FUNCTION_BLOCK "IMAC_VALVE"
TITLE = VALVE
//--------------------------------------------------------------------------------
//SIEMENS AG     I&S IP PEP SN                       PSP-Element: D-09300081-E-E5
//--------------------------------------------------------------------------------
//History
//=======
//Date       Version Description                     Author
//1997/06/09   0.6   Basic EditionHeino              Salge
//2004/11/05   1.0   Basic Edition converted to S7   Edelmann
//2004/12/07   1.1   Interface adapted               Edelmann
//2004/12/16   1.2   ACOM converted to WORD          Edelmann
//
//--------------------------------------------------------------------------------
//PLC:   >= S7-300
//--------------------------------------------------------------------------------
//Specification:   Refer "TECHFUNK.DOC"
//--------------------------------------------------------------------------------
//Called FC: FC90 "DELAYTIMER"
//           SFC20 "BLKMOV"
//--------------------------------------------------------------------------------
//at run time:
//--------------------------------------------------------------------------------
//
//--------------------------------------------------------------------------------
//Note:
//--------------------------------------------------------------------------------
// KNOW_HOW_PROTECT
AUTHOR : Sa_Edm
FAMILY : IMAC
NAME : VALVE
VERSION : 1.2


VAR_INPUT
  OBJ : INT ;
  RMOT : BOOL ;	//Local / Remote
  OPEN : BOOL ;
  CLSD : BOOL ;
  ACOM : WORD ;
  FAUL : BOOL ;
  PCONF : STRUCT
   LastRecord : INT  := 100;
   Pointer1stRecord : STRUCT
    S7ID : BYTE  := B#16#10;	//ANY pointer: ID S7
    Typ : BYTE  := B#16#2;	//ANY pointer: data typ =02 BYTE =04 WORD =05 INT =06 DWORD =07 DINT =08 REAL
    RepeatFactor : INT  := 104;	//ANY pointer: repeat factor
    DBNo : INT  := 83;	//ANY pointer: DB number, zero if no DB
    MemoryArea : BYTE  := B#16#84;	//ANY pointer: Memory area =81 IN =82 OUT =83 M =84 DB =85 DI =86 L
    DWHigh : BYTE ;	//ANY pointer: DW highest byte
    DWX : INT ;	//ANY pointer: DW low / bit (address = byte *8 + bit)
   END_STRUCT ;
  END_STRUCT ;
END_VAR
VAR_OUTPUT
  VOPN : BOOL ;
  VCLS : BOOL ;
  STAT : WORD ;
  OSSTAT : WORD ;	//Status for OS
  OSALARM : WORD ;	//Alarms for OS
END_VAR
VAR_IN_OUT
  OSCOM : WORD ;
END_VAR
VAR
  VALVE : STRUCT
   System : WORD ;
   CmdOS : WORD ;
   MirrorCmdOS : WORD ;
   Test : WORD ;
   AlarmOS : WORD ;
   StatusOS : WORD ;
   SysStatusOS : WORD ;
   Status1 : WORD ;
   Status2 : WORD ;
   Status3 : BYTE ;
   InputEdges : BYTE ;
   AutoEdges : WORD ;
   DataTimeActFault : STRUCT
    StartTime : DINT ;
    StartEdge : BOOL ;
   END_STRUCT ;
   DataTimeOpening : STRUCT
    StartTime : DINT ;
    StartEdge : BOOL ;
   END_STRUCT ;
   DataTimeClosing : STRUCT
    StartTime : DINT ;
    StartEdge : BOOL ;
   END_STRUCT ;
   DataTimeFeedback : STRUCT
    StartTime : DINT ;
    StartEdge : BOOL ;
   END_STRUCT ;
   DataTimeReverse : STRUCT
    StartTime : DINT ;
    StartEdge : BOOL ;
   END_STRUCT ;
   DataTimeOvertravel : STRUCT
    StartTime : DINT ;
    StartEdge : BOOL ;
   END_STRUCT ;
   DataTimeExtFault : STRUCT
    StartTime : DINT ;
    StartEdge : BOOL ;
   END_STRUCT ;
   DataTimeRestart : STRUCT
    StartTime : DINT ;
    StartEdge : BOOL ;
   END_STRUCT ;
   PCONF : STRUCT
    Modeswitches : STRUCT
     M0_SingleActingValve : BOOL ;	// Single acting valve (1); Double acting valve (0)
     M1_ResetMode : BOOL ;	// Open/Close and RESET (1); only RESET (0)
     M2_OperationMode : BOOL ;	// AUTO/MANUAL/LOCAL(1); Only MANUAL/LOCAL
     M3_Status : BOOL ;	// Change status OPENED/CLOSED by switching from REMOTE to LOCAL (1)
     M4_LockInput : BOOL ;	// Commands and failure (1); only failure
     M5_ESO : BOOL ;	// Open valve if ESO=1 (1); Close valve if ESO=1 (0)
     M6_ReverseTime : BOOL ;	// Double acting valves: Reverse Time ON
     M7_OvertravelTime : BOOL ;	// Double acting valves: Overtravel Time ON
     M8_Spare : BOOL ;	// Spare
     M9_OpenAfterBlackout : BOOL ;	// Open after blackout (1)
     M10_ExtFaultNC : BOOL ;	// External Fault is NC (1); NO (0)
     M11_Spare : BOOL ;	// Spare
     M12_Spare : BOOL ;	// Spare
     M13_LocalAutoMode : BOOL ;	// Set automatic status if RMOT-input is in local
     M14_Spare : BOOL ;	// Spare
     M15_Test : BOOL ;	// Testbit (1)
    END_STRUCT ;
    DlyTActFault : TIME ;	// Setpoint Action Fault delay
    DlyTOpening : TIME ;	// Setpoint Waiting Delay Slow->Fast
    DlyTClosing : TIME ;	// Setpoint Waiting Delay Fast->Slow
    DlyTFeedback : TIME ;	// Setpoint feedback fault delay
    DlyTReverse : TIME ;	// Setpoint change direction
    DlyTOvertravel : TIME ;	// Setpoint auto alarm delay
    DlyTExtFault : TIME ;	// Setpoint external fault delay
    DlyTRestart : TIME ;	// Setpoint restart after blackout delay
   END_STRUCT ;
  END_STRUCT ;
  siFailRR : INT ;	//Falure blockmove readrecord
  siFailWR : INT ;	//Failure blokmove write record
END_VAR
VAR_TEMP
  M200_0 : BOOL ;
  tbCmdManual : BOOL ;
  tbCmdAuto : BOOL ;
  M200_3 : BOOL ;
  M200_4 : BOOL ;
  M200_5 : BOOL ;
  M200_6 : BOOL ;
  M200_7 : BOOL ;
  tbOSCmdOpen : BOOL ;
  tbOSCmdClose : BOOL ;
  tbOSCmdTgOpCl : BOOL ;
  M201_3 : BOOL ;
  M201_4 : BOOL ;
  M201_5 : BOOL ;
  M201_6 : BOOL ;
  tbCmdReset : BOOL ;
  M202_0 : BOOL ;
  M202_1 : BOOL ;
  M202_2 : BOOL ;
  M202_3 : BOOL ;
  M202_4 : BOOL ;
  M202_5 : BOOL ;
  M202_6 : BOOL ;
  M202_7 : BOOL ;
  M203_0 : BOOL ;
  M203_1 : BOOL ;
  M203_2 : BOOL ;
  tbLock : BOOL ;
  tbAmergency : BOOL ;
  tbBlackout : BOOL ;
  tb24VPleiger : BOOL ;
  M203_7 : BOOL ;
  M204_0 : BOOL ;
  M204_1 : BOOL ;
  M204_2 : BOOL ;
  M204_3 : BOOL ;
  M204_4 : BOOL ;
  M204_5 : BOOL ;
  M204_6 : BOOL ;
  M204_7 : BOOL ;
  tbCmdOpenAuto : BOOL ;
  tbCmdCloseAuto : BOOL ;
  M205_2 : BOOL ;
  M205_3 : BOOL ;
  M205_4 : BOOL ;
  M205_5 : BOOL ;
  M205_6 : BOOL ;
  M205_7 : BOOL ;
  tbRemote : BOOL ;
  tbOpen : BOOL ;
  tbClosed : BOOL ;
  tbFault : BOOL ;
  M206_4 : BOOL ;
  M206_5 : BOOL ;
  M206_6 : BOOL ;
  tbLocal : BOOL ;
  M207_0 : BOOL ;
  M207_1 : BOOL ;
  M207_2 : BOOL ;
  M207_3 : BOOL ;
  M207_4 : BOOL ;
  M207_5 : BOOL ;
  M207_6 : BOOL ;
  M207_7 : BOOL ;
  M208_0 : BOOL ;
  M208_1 : BOOL ;
  M208_2 : BOOL ;
  M208_3 : BOOL ;
  M208_4 : BOOL ;
  M208_5 : BOOL ;
  M208_6 : BOOL ;
  M208_7 : BOOL ;
  tbStateOpen : BOOL ;
  tbStateClosed : BOOL ;
  tbStateLocal : BOOL ;
  tbStateManual : BOOL ;
  tbStateAuto : BOOL ;
  tbStateOpening : BOOL ;
  tbStateClosing : BOOL ;
  tbStateAlarm : BOOL ;
  M210_0 : BOOL ;
  M210_1 : BOOL ;
  M210_2 : BOOL ;
  M210_3 : BOOL ;
  M210_4 : BOOL ;
  M210_5 : BOOL ;
  M210_6 : BOOL ;
  M210_7 : BOOL ;
  M211_0 : BOOL ;
  M211_1 : BOOL ;
  M211_2 : BOOL ;
  M211_3 : BOOL ;
  M211_4 : BOOL ;
  M211_5 : BOOL ;
  M211_6 : BOOL ;
  M211_7 : BOOL ;
  M212_0 : BOOL ;
  M212_1 : BOOL ;
  M212_2 : BOOL ;
  M212_3 : BOOL ;
  M212_4 : BOOL ;
  M212_5 : BOOL ;
  M212_6 : BOOL ;
  M212_7 : BOOL ;
  M213_0 : BOOL ;
  M213_1 : BOOL ;
  M213_2 : BOOL ;
  M213_3 : BOOL ;
  M213_4 : BOOL ;
  M213_5 : BOOL ;
  M213_6 : BOOL ;
  M213_7 : BOOL ;
  tbRstClsTimer : BOOL ;
  tbRstClsAlarm : BOOL ;
  tbRstFBTimer : BOOL ;
  tbRstFBAlarm : BOOL ;
  tbRstRevTimer : BOOL ;
  tbRstOvertrTimer : BOOL ;
  tbRstFaultTimer : BOOL ;
  tbExtFault : BOOL ;
  tbOutOpen : BOOL ;
  tbOutClose : BOOL ;
  tbOutManual : BOOL ;
  tbOutAuto : BOOL ;
  tbRstActTimer : BOOL ;
  tbRstActAlarm : BOOL ;
  tbRstOpnTimer : BOOL ;
  tbRstOpnAlarm : BOOL ;
  tbVOPN : BOOL ;
  tbVCLS : BOOL ;
  M216_2 : BOOL ;
  M216_3 : BOOL ;
  M216_4 : BOOL ;
  M216_5 : BOOL ;
  M216_6 : BOOL ;
  M216_7 : BOOL ;
  tbReverseCopen : BOOL ;
  tbReverseClose : BOOL ;
  tbOpenAfterBO : BOOL ;
  tbBOTimerActiv : BOOL ;
  M217_4 : BOOL ;
  M217_5 : BOOL ;
  M217_6 : BOOL ;
  M217_7 : BOOL ;
  tbLocalToRemote : BOOL ;
  tbOpenPulse : BOOL ;
  M218_2 : BOOL ;
  M218_3 : BOOL ;
  M218_4 : BOOL ;
  M218_5 : BOOL ;
  M218_6 : BOOL ;
  tbchgeRemLoc : BOOL ;
  M219_0 : BOOL ;
  M219_1 : BOOL ;
  tbClosePulse : BOOL ;
  M219_3 : BOOL ;
  M219_4 : BOOL ;
  M219_5 : BOOL ;
  M219_6 : BOOL ;
  M219_7 : BOOL ;
  M220_0 : BOOL ;
  M220_1 : BOOL ;
  M220_2 : BOOL ;
  M220_3 : BOOL ;
  M220_4 : BOOL ;
  M220_5 : BOOL ;
  M220_6 : BOOL ;
  M220_7 : BOOL ;
  M221_0 : BOOL ;
  M221_1 : BOOL ;
  M221_2 : BOOL ;
  M221_3 : BOOL ;
  M221_4 : BOOL ;
  M221_5 : BOOL ;
  M221_6 : BOOL ;
  M221_7 : BOOL ;
  P_currentRecord : ANY ;	//ANY pointer of the current record
END_VAR
BEGIN
NETWORK
TITLE =Calculation of current ANY pointer for reading /writing record
// ANY-pointer of current record
      L     #PCONF.Pointer1stRecord.S7ID;
      T     LB    22;
      L     #PCONF.Pointer1stRecord.Typ;
      T     LB    23;
      L     #PCONF.Pointer1stRecord.RepeatFactor;
      T     LW    24;
      L     #PCONF.Pointer1stRecord.DBNo;
      T     LW    26;
      L     #PCONF.Pointer1stRecord.MemoryArea;
      T     LB    28;
      L     #PCONF.Pointer1stRecord.DWHigh;
      T     LB    29;
      L     #PCONF.Pointer1stRecord.DWX;
      T     LW    30;

      L     #OBJ; //Check whether Obj within the range
      L     #PCONF.LastRecord;
      >I    ;
      SPB   cRcd;
      L     #OBJ;
      L     1;
      <I    ;
      SPB   cRcd;
      L     #OBJ;
cRcd: +     -1;
      L     #PCONF.Pointer1stRecord.RepeatFactor;
      *I    ;
      SLD   3; //DBW + DBX address of the current record
      L     LD    28;
      OD    ;
      T     LD    28; //DBWX part of ANY pointer "P_currentRecord"

NETWORK
TITLE =Read record

      CALL "BLKMOV" (
           SRCBLK                   := #P_currentRecord,
           RET_VAL                  := #siFailRR,
           DSTBLK                   := #VALVE);

NETWORK
TITLE =Read OS command

      L     #OSCOM; // Commands from OS
      T     LW     0;
      L     #VALVE.Status1; // Status stored
      T     LW    14;
      L     #VALVE.Status2; // Status stored
      T     LW    16;

      L     0; //Reset scratch  flags
      T     LW     6;
      T     LW    50;
      T     LW    52;
      T     LW    54;
NETWORK
TITLE =Formaloperanden Inputs

      U     #RMOT;
      =     #tbRemote; // Remote
      U     #OPEN;
      =     #tbOpen; // OPEN
      U     #CLSD;
      =     #tbClosed; // CLOSED


      U     #VALVE.PCONF.Modeswitches.M10_ExtFaultNC;
      SPB   NC; //jump Normal Closed Input
      U     #FAUL;
      =     #tbFault; // Fault
      SPA   GO;
NC:   UN    #FAUL;
      =     #tbFault; // Fault

GO:   L     #ACOM;
      T     LW     2;

      UN    #tbRemote; // Not Remote
      =     #tbLocal; // Local

// ----Evaluate Pulsflags from Auto Commands----
      L     #VALVE.AutoEdges; //Stored Auto Command last cycle
      INVI  ; //Singlecomplement
      L     LW     2; //Command From Automatic
      T     #VALVE.AutoEdges;
      UW    ;
      T     LW     4; // Command  Pulseflags

// ----Evaluate Pulsflags from Inputs----
      L     #VALVE.InputEdges; //Stored Auto Command last cycle
      INVI  ; //Singlecomplement
      L     LB     6; //Inputs
      T     #VALVE.InputEdges;
      UW    ;
      T     LB    18; // Inputs Pulseflags
NETWORK
TITLE =Local-Manual- Auto

      U     #VALVE.PCONF.Modeswitches.M13_LocalAutoMode; // Modeswitch Autostatus if RMOT INPUT in Local
      SPB   LoAu;

      U     #tbRemote; // Remote
      SPB   RMOT;

      R     #tbOutManual; // MANUAL!
      R     #tbOutAuto; // AUTO!
      R     #tbRstActTimer; // reset Action Timer
      R     #tbRstOpnTimer; // reset Opening Alarm timer
      R     #tbRstClsTimer; // reset Closing Alarm timer
      R     #tbRstFBTimer; // reset Non-Feedback timer
      R     #tbRstRevTimer; // reset Reverse timer
      R     #tbRstOvertrTimer; // reset Overtravel timer
      R     #tbOpenAfterBO; // Open after Blackout

      UN    #VALVE.PCONF.Modeswitches.M3_Status; // Modeswitch Change Open Close If Remote-Local
      R     #tbOutOpen; // OPEN!
      R     #tbOutClose; // CLOSE!
      SPB   E5;

      U     #tbchgeRemLoc; // Change from Remote to Local Pulse
      U     #tbOutOpen; // OPEN!
      R     #tbOutOpen; // OPEN!
      S     #tbOutClose; // CLOSE!
      SPB   E5;

      U     #tbchgeRemLoc; // Change from Remote to Local Pulse
      U     #tbOutClose; // CLOSE!
      R     #tbOutClose; // CLOSE!
      S     #tbOutOpen; // OPEN!
      SPA   E5;

RMOT: U     #VALVE.PCONF.Modeswitches.M2_OperationMode; // extra Automode ?
      SPB   MODE;
      S     #tbOutManual; // MANUAL!
      S     #tbOutAuto; // AUTO!
      SPA   E5;

MODE: U     #tbCmdManual; // Command Manual
      S     #tbOutManual; // MANUAL!
      R     #tbOutAuto; // AUTO!
      U     #tbCmdAuto; // Command Auto
      S     #tbOutAuto; // AUTO!
      R     #tbOutManual; // MANUAL!
      UN    #tbOutAuto; // AUTO!
      UN    #tbOutManual; // MANUAL!
      S     #tbOutManual; // MANUAL!
      SPA   E5;

LoAu: U     #tbLocal; // Local
      S     #tbOutAuto; // AUTO!
      R     #tbOutManual; // MANUAL!
      U     #tbRemote; // Remote
      R     #tbOutAuto; // AUTO!
      S     #tbOutManual; // MANUAL!

E5:   NOP   0;
NETWORK
TITLE =Commands
//-------SET OpenCommand----------
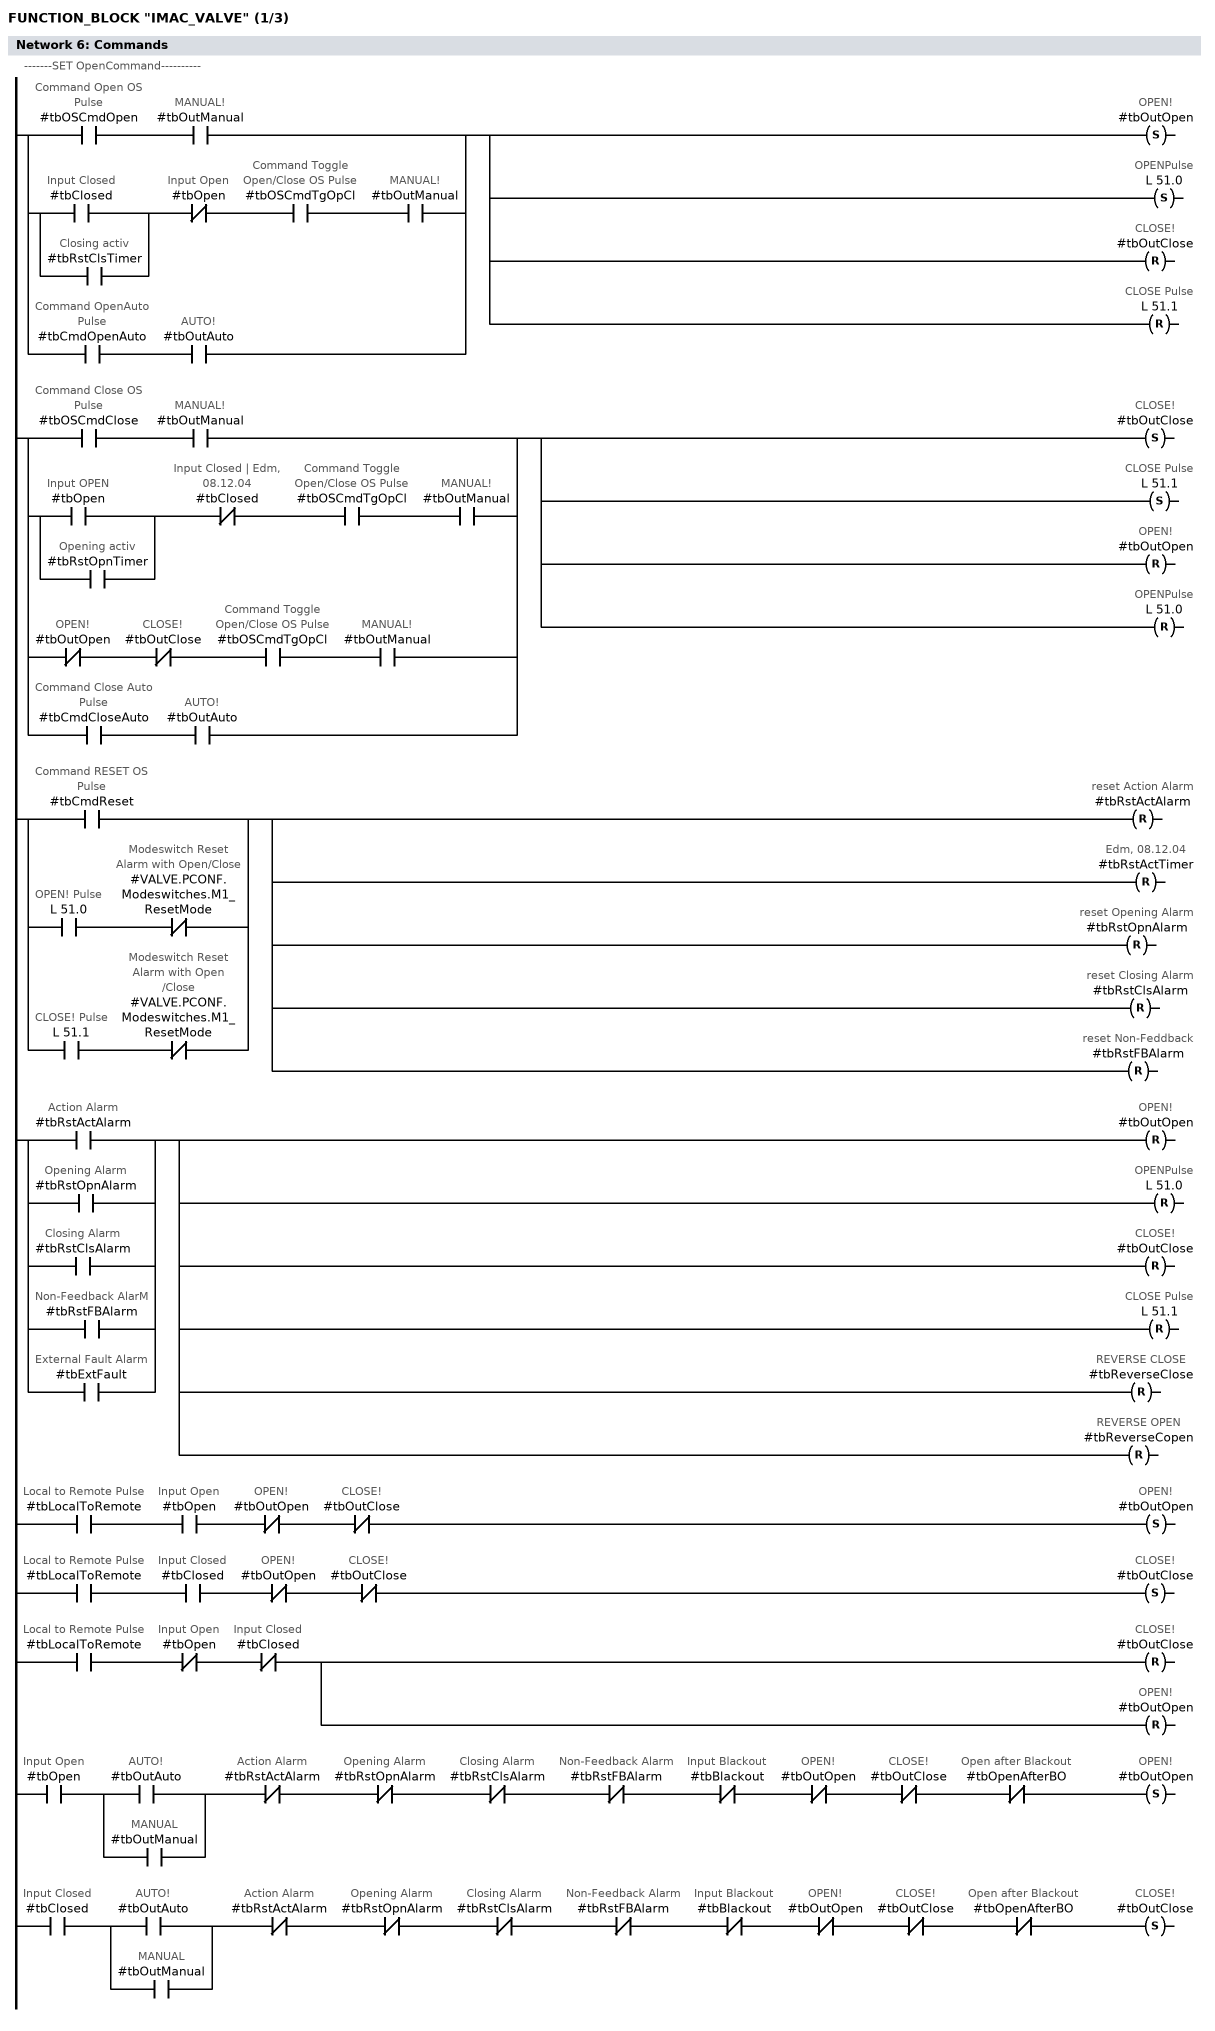
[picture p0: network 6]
      O(    ;
      U     #tbOSCmdOpen; //Command Open OS Pulse
      U     #tbOutManual; // MANUAL!
      )     ;
      O(    ;
      O     #tbClosed; // Input Closed
      O     #tbRstClsTimer; // Closing activ
      UN    #tbOpen; // Input Open
      U     #tbOSCmdTgOpCl; // Command Toggle Open/Close OS Pulse
      U     #tbOutManual; // MANUAL!
      )     ;
      O(    ;
      U     #tbCmdOpenAuto; //Command OpenAuto Pulse
      U     #tbOutAuto; // AUTO!
      )     ;
      S     #tbOutOpen; // OPEN!
      S     L     51.0; // OPENPulse
      R     #tbOutClose; // CLOSE!
      R     L     51.1; // CLOSE Pulse

//-------SET Close Command----------
      O(    ;
      U     #tbOSCmdClose; //Command Close OS Pulse
      U     #tbOutManual; // MANUAL!
      )     ;
      O(    ;
      O     #tbOpen; // Input OPEN
      O     #tbRstOpnTimer; // Opening activ
      UN    #tbClosed; // Input Closed | Edm, 08.12.04
      U     #tbOSCmdTgOpCl; // Command Toggle Open/Close OS Pulse
      U     #tbOutManual; // MANUAL!
      )     ;
      O(    ;
      UN    #tbOutOpen; // OPEN!
      UN    #tbOutClose; // CLOSE!
      U     #tbOSCmdTgOpCl; // Command Toggle Open/Close OS Pulse
      U     #tbOutManual; // MANUAL!
      )     ;
      O(    ;
      U     #tbCmdCloseAuto; //Command Close Auto Pulse
      U     #tbOutAuto; // AUTO!
      )     ;
      S     #tbOutClose; // CLOSE!
      S     L     51.1; // CLOSE Pulse
      R     #tbOutOpen; // OPEN!
      R     L     51.0; // OPENPulse

//-------Reset Alarms----------
      O     #tbCmdReset; //Command RESET OS Pulse
      O(    ;
      U     L     51.0; // OPEN! Pulse
      UN    #VALVE.PCONF.Modeswitches.M1_ResetMode; // Modeswitch Reset Alarm with Open/Close
      )     ;
      O(    ;
      U     L     51.1; // CLOSE! Pulse
      UN    #VALVE.PCONF.Modeswitches.M1_ResetMode; // Modeswitch Reset Alarm with Open /Close
      )     ;
      R     #tbRstActAlarm; // reset Action Alarm
      R     #tbRstActTimer; // Edm, 08.12.04
      R     #tbRstOpnAlarm; // reset Opening Alarm
      R     #tbRstClsAlarm; // reset Closing Alarm
      R     #tbRstFBAlarm; // reset Non-Feddback


//-------Reset Commands----------
      O     #tbRstActAlarm; // Action Alarm
      O     #tbRstOpnAlarm; // Opening Alarm
      O     #tbRstClsAlarm; // Closing Alarm
      O     #tbRstFBAlarm; // Non-Feedback AlarM
      O     #tbExtFault; // External Fault Alarm
      R     #tbOutOpen; // OPEN!
      R     L     51.0; // OPENPulse
      R     #tbOutClose; // CLOSE!
      R     L     51.1; // CLOSE Pulse
      R     #tbReverseClose; // REVERSE CLOSE
      R     #tbReverseCopen; // REVERSE OPEN

//-------Local Remote change ----------
      U     #tbLocalToRemote; // Local to Remote Pulse
      U     #tbOpen; // Input Open
      UN    #tbOutOpen; // OPEN!
      UN    #tbOutClose; // CLOSE!
      S     #tbOutOpen; // OPEN!

      U     #tbLocalToRemote; // Local to Remote Pulse
      U     #tbClosed; // Input Closed
      UN    #tbOutOpen; // OPEN!
      UN    #tbOutClose; // CLOSE!
      S     #tbOutClose; // CLOSE!

      U     #tbLocalToRemote; // Local to Remote Pulse
      UN    #tbOpen; // Input Open
      UN    #tbClosed; // Input Closed
      R     #tbOutClose; // CLOSE!
      R     #tbOutOpen; // OPEN!

//-------Set State after Failure or Blackout if Remote----------
      U     #tbOpen; // Input Open
      U(    ;
      O     #tbOutAuto; // AUTO!
      O     #tbOutManual; // MANUAL
      )     ;
      UN    #tbRstActAlarm; // Action Alarm
      UN    #tbRstOpnAlarm; // Opening Alarm
      UN    #tbRstClsAlarm; // Closing Alarm
      UN    #tbRstFBAlarm; // Non-Feedback Alarm
      UN    #tbBlackout; // Input Blackout
      UN    #tbOutOpen; // OPEN!
      UN    #tbOutClose; // CLOSE!
      UN    #tbOpenAfterBO; // Open after Blackout
      S     #tbOutOpen; // OPEN!

      U     #tbClosed; // Input Closed
      U(    ;
      O     #tbOutAuto; // AUTO!
      O     #tbOutManual; // MANUAL
      )     ;
      UN    #tbRstActAlarm; // Action Alarm
      UN    #tbRstOpnAlarm; // Opening Alarm
      UN    #tbRstClsAlarm; // Closing Alarm
      UN    #tbRstFBAlarm; // Non-Feedback Alarm
      UN    #tbBlackout; // Input Blackout
      UN    #tbOutOpen; // OPEN!
      UN    #tbOutClose; // CLOSE!
      UN    #tbOpenAfterBO; // Open after Blackout
      S     #tbOutClose; // CLOSE!
NETWORK
TITLE =OPEN after Blackout
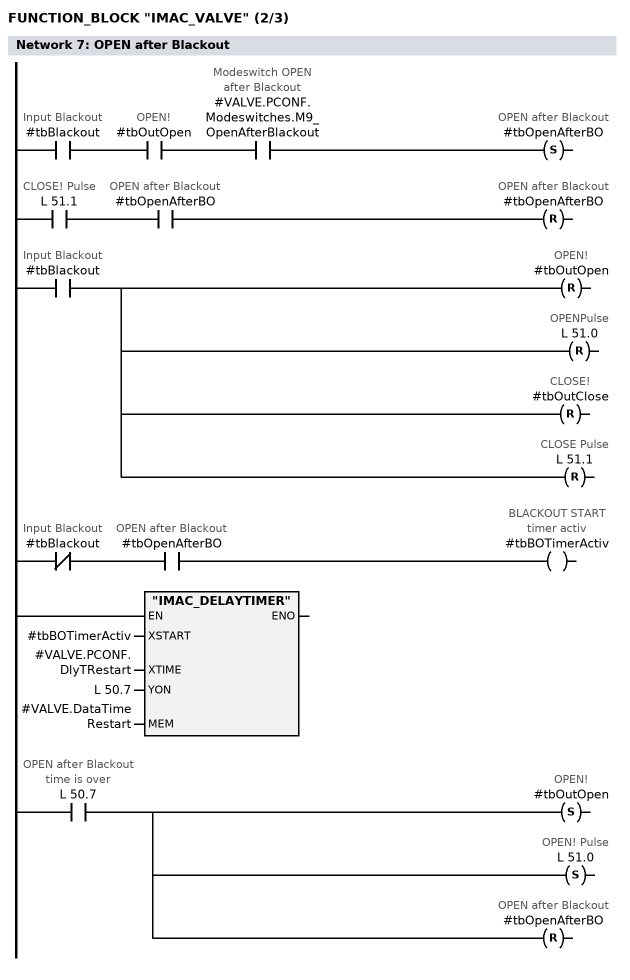
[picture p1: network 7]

      U     #tbBlackout; // Input Blackout
      U     #tbOutOpen; // OPEN!
      U     #VALVE.PCONF.Modeswitches.M9_OpenAfterBlackout; // Modeswitch OPEN after Blackout
      S     #tbOpenAfterBO; // OPEN after Blackout

      U     L     51.1; // CLOSE! Pulse
      U     #tbOpenAfterBO; // OPEN after Blackout
      R     #tbOpenAfterBO; // OPEN after Blackout

      U     #tbBlackout; // Input Blackout
      R     #tbOutOpen; // OPEN!
      R     L     51.0; // OPENPulse
      R     #tbOutClose; // CLOSE!
      R     L     51.1; // CLOSE Pulse

      UN    #tbBlackout; // Input Blackout
      U     #tbOpenAfterBO; // OPEN after Blackout
      =     #tbBOTimerActiv; // BLACKOUT START timer activ

//Blackout recovery timer
      CALL "IMAC_DELAYTIMER" (
           XSTART                   := #tbBOTimerActiv,// BLACKOUT START timer activ
           XTIME                    := #VALVE.PCONF.DlyTRestart,
           YON                      := L     50.7,
           MEM                      := #VALVE.DataTimeRestart);

      U     L     50.7; // OPEN after Blackout time is over
      S     #tbOutOpen; // OPEN!
      S     L     51.0; // OPEN! Pulse
      R     #tbOpenAfterBO; // OPEN after Blackout
NETWORK
TITLE =Action Alarm
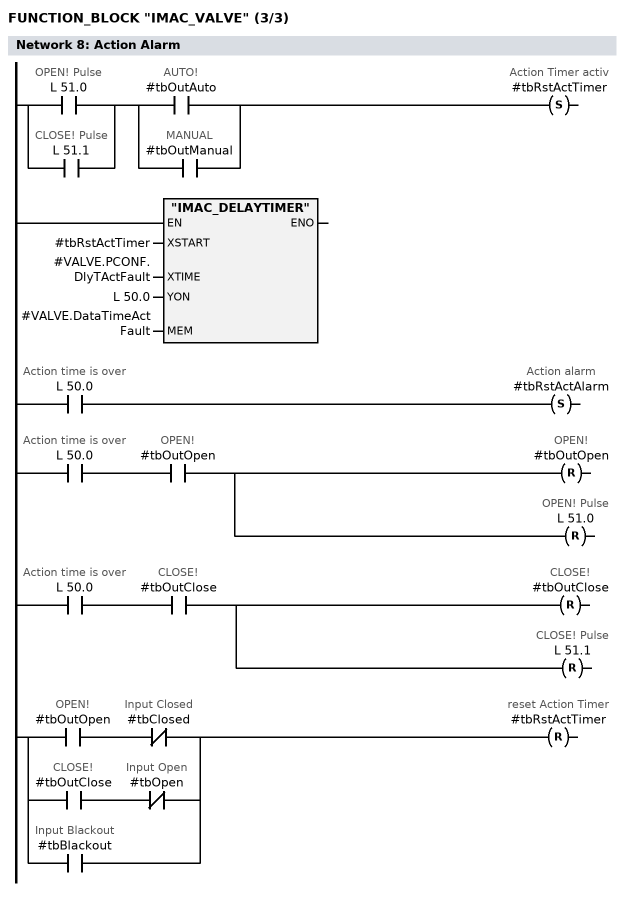
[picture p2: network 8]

      O     L     51.0; // OPEN! Pulse
      O     L     51.1; // CLOSE! Pulse
      U(    ;
      O     #tbOutAuto; // AUTO!
      O     #tbOutManual; // MANUAL
      )     ;
      S     #tbRstActTimer; // Action Timer activ

//Action timer
      CALL "IMAC_DELAYTIMER" (
           XSTART                   := #tbRstActTimer,//Action Timer activ
           XTIME                    := #VALVE.PCONF.DlyTActFault,
           YON                      := L     50.0,
           MEM                      := #VALVE.DataTimeActFault);

      U     L     50.0; // Action time is over
      S     #tbRstActAlarm; // Action alarm

      U     L     50.0; // Action time is over
      U     #tbOutOpen; // OPEN!
      R     #tbOutOpen; // OPEN!
      R     L     51.0; // OPEN! Pulse

      U     L     50.0; // Action time is over
      U     #tbOutClose; // CLOSE!
      R     #tbOutClose; // CLOSE!
      R     L     51.1; // CLOSE! Pulse

      O(    ;
      U     #tbOutOpen; // OPEN!
      UN    #tbClosed; // Input Closed
      )     ;
      O(    ;
      U     #tbOutClose; // CLOSE!
      UN    #tbOpen; // Input Open
      )     ;
      O     #tbBlackout; // Input Blackout
      R     #tbRstActTimer; // reset Action Timer



NETWORK
TITLE =Overtravel timer

      UN    #tbOutAuto; // AUTO!
      UN    #tbOutManual; // MANUAL
      ON    #VALVE.PCONF.Modeswitches.M7_OvertravelTime; // Modeswitch Overtravel timer
      SPB   E9;

      O(    ;
      U     #tbOutOpen; // OPEN!
      U     #tbRstOpnTimer; // Opening activ
      U     #tbOpenPulse; // Input Open Pulse
      )     ;
      O(    ;
      U     #tbOutClose; // CLOSE!
      U     #tbRstClsTimer; // Closing timer activ
      U     #tbClosePulse; // Input Closed pulse
      )     ;
      S     #tbRstOvertrTimer; // Overtravel timer activ

//Change direction timer
      CALL "IMAC_DELAYTIMER" (
           XSTART                   := #tbRstOvertrTimer,//Change direction time
           XTIME                    := #VALVE.PCONF.DlyTOvertravel,
           YON                      := L     50.6,
           MEM                      := #VALVE.DataTimeOvertravel);

      O     L     50.6; // Overtravel timer is over
      O     #tbBlackout; // Input Blackout
      R     #tbRstOvertrTimer; // Overtravel timer activ
E9:   NOP   0;

NETWORK
TITLE =Reverse Timer

      UN    #tbOutAuto; // AUTO!
      UN    #tbOutManual; // MANUAL
      ON    #VALVE.PCONF.Modeswitches.M6_ReverseTime; // Modeswitch Reverse Time
      SPB   E10;
      U     #tbRstOpnTimer; // Opening activ
      U     L     51.1; // CLOSE! Pulse
      S     #tbReverseClose; // REVERSE CLOSE
      R     #tbReverseCopen; // REVERSE OPEN
      R     #tbOutClose; // CLOSE!
      R     L     51.1; // CLOSE! Pulse
      R     #tbRstOpnTimer; // Opening activ

      U     #tbRstClsTimer; // Closing activ
      U     L     51.0; // OPEN! Pulse
      S     #tbReverseCopen; // REVERSE OPEN
      R     #tbReverseClose; // REVERSE CLOSE
      R     #tbOutOpen; // OPEN!
      R     L     51.0; // OPEN! Pulse
      R     #tbRstClsTimer; // Closing activ

      U     L     51.0; // OPEN! Pulse
      U     #tbReverseClose; // REVERSE CLOSE
      S     #tbReverseCopen; // REVERSE OPEN
      R     #tbReverseClose; // REVERSE CLOSE
      R     #tbOutOpen; // OPEN!
      R     L     51.0; // OPEN! Pulse

      U     L     51.1; // CLOSE! Pulse
      U     #tbReverseCopen; // REVERSE OPEN
      S     #tbReverseClose; // REVERSE CLOSE
      R     #tbReverseCopen; // REVERSE OPEN
      R     #tbOutClose; // CLOSE!
      R     L     51.1; // CLOSE! Pulse

      O     #tbReverseClose; // REVERSE CLOSE
      O     #tbReverseCopen; // REVERSE OPEN
      S     #tbRstRevTimer; // Reverse Timer activ

//Reverse timer
      CALL "IMAC_DELAYTIMER" (
           XSTART                   := #tbRstRevTimer,//Reverse Timer activ
           XTIME                    := #VALVE.PCONF.DlyTReverse,
           YON                      := L     50.5,
           MEM                      := #VALVE.DataTimeReverse);

      U     L     50.5; // Reverse time is over
      U     #tbReverseCopen; // Reverse Open
      S     #tbOutOpen; // OPEN!
      S     L     51.0; // OPEN! Pulse
      R     #tbRstRevTimer; // Reverse Timer activ
      R     #tbReverseCopen; // REVERSE OPEN

      U     L     50.5; // Reverse time is over
      U     #tbReverseClose; // REVERSE CLOSE
      S     #tbOutClose; // CLOSE!
      S     L     51.1; // CLOSE! Pulse
      R     #tbRstRevTimer; // Reverse Timer activ
      R     #tbReverseClose; // REVERSE CLOSE

      O     #tbBlackout; // Input Blackout
      R     #tbRstRevTimer; // Reverse Timer activ
      R     #tbReverseClose; // REVERSE CLOSE
      R     #tbReverseCopen; // REVERSE OPEN

E10:  NOP   0;
NETWORK
TITLE =Opening / Closing Alarm
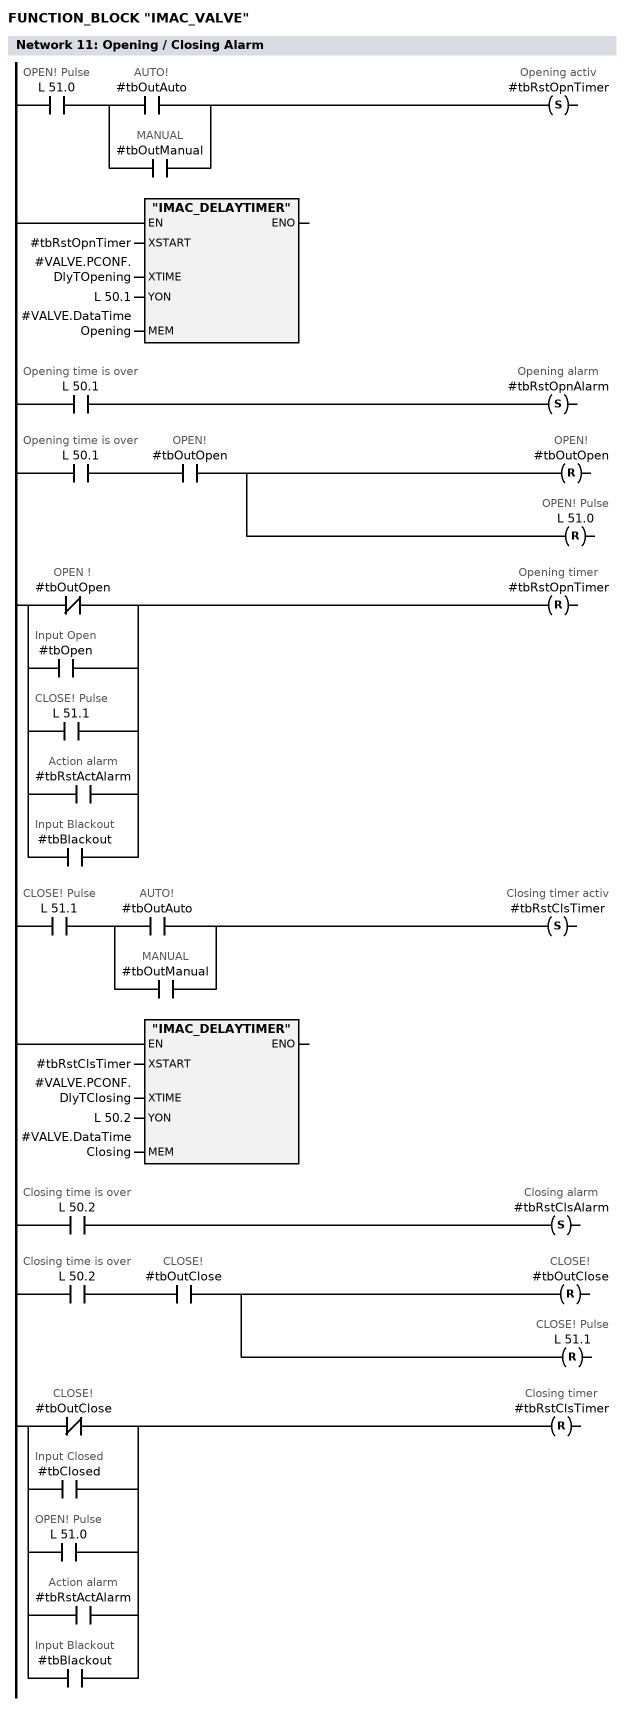
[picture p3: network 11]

      U     L     51.0; // OPEN! Pulse
      U(    ;
      O     #tbOutAuto; // AUTO!
      O     #tbOutManual; // MANUAL
      )     ;
      S     #tbRstOpnTimer; // Opening activ

//Opening timer
      CALL "IMAC_DELAYTIMER" (
           XSTART                   := #tbRstOpnTimer,//Opening timer activ
           XTIME                    := #VALVE.PCONF.DlyTOpening,
           YON                      := L     50.1,
           MEM                      := #VALVE.DataTimeOpening);

      U     L     50.1; // Opening time is over
      S     #tbRstOpnAlarm; // Opening alarm
      U     L     50.1; // Opening time is over
      U     #tbOutOpen; // OPEN!
      R     #tbOutOpen; // OPEN!
      R     L     51.0; // OPEN! Pulse

      ON    #tbOutOpen; // OPEN !
      O     #tbOpen; // Input Open
      O     L     51.1; // CLOSE! Pulse
      O     #tbRstActAlarm; // Action alarm
      O     #tbBlackout; // Input Blackout
      R     #tbRstOpnTimer; // Opening timer


      O     L     51.1; // CLOSE! Pulse
      U(    ;
      O     #tbOutAuto; // AUTO!
      O     #tbOutManual; // MANUAL
      )     ;
      S     #tbRstClsTimer; // Closing timer activ

//Closing timer
      CALL "IMAC_DELAYTIMER" (
           XSTART                   := #tbRstClsTimer,//Closing time
           XTIME                    := #VALVE.PCONF.DlyTClosing,
           YON                      := L     50.2,
           MEM                      := #VALVE.DataTimeClosing);

      U     L     50.2; // Closing time is over
      S     #tbRstClsAlarm; // Closing alarm
      U     L     50.2; // Closing time is over
      U     #tbOutClose; // CLOSE!
      R     #tbOutClose; // CLOSE!
      R     L     51.1; // CLOSE! Pulse

      ON    #tbOutClose; // CLOSE!
      O     #tbClosed; // Input Closed
      O     L     51.0; // OPEN! Pulse
      O     #tbRstActAlarm; // Action alarm
      O     #tbBlackout; // Input Blackout
      R     #tbRstClsTimer; // Closing timer


NETWORK
TITLE =External Fault Alarm

      O     #tbOutAuto; // AUTO!
      O     #tbOutManual; // MANUAL!
      SPB   RMO1;
      U     #tbFault; // External Fault
      =     #tbExtFault; // External Fault Alarm
      R     #tbOutOpen; // OPEN!
      R     L     51.0; // OPEN! Pulse
      R     #tbOutClose; // CLOSE!
      R     L     51.1; // CLOSE! Pulse
      SPA   E12;
RMO1: U     #tbFault; // External Fault
      UN    #tbExtFault; // External Fault Alarm
      UN    #tbBlackout; // Blackout
      =     #tbRstFaultTimer; // Fault timer activ

//Fault timer
      CALL "IMAC_DELAYTIMER" (
           XSTART                   := #tbRstFaultTimer,// Fault timer activ
           XTIME                    := #VALVE.PCONF.DlyTExtFault,
           YON                      := L     50.3,
           MEM                      := #VALVE.DataTimeExtFault);

      U     L     50.3; // Fault time over
      S     #tbExtFault; // External Fault Alarm
      R     #tbOutOpen; // OPEN!
      R     L     51.0; // OPEN! Pulse
      R     #tbOutClose; // CLOSE!
      R     L     51.1; // CLOSE! Pulse
      UN    #tbFault; // External Fault
      R     #tbExtFault; // External Fault Alarm
E12:  NOP   0;
NETWORK
TITLE =Non-Feedback alarm
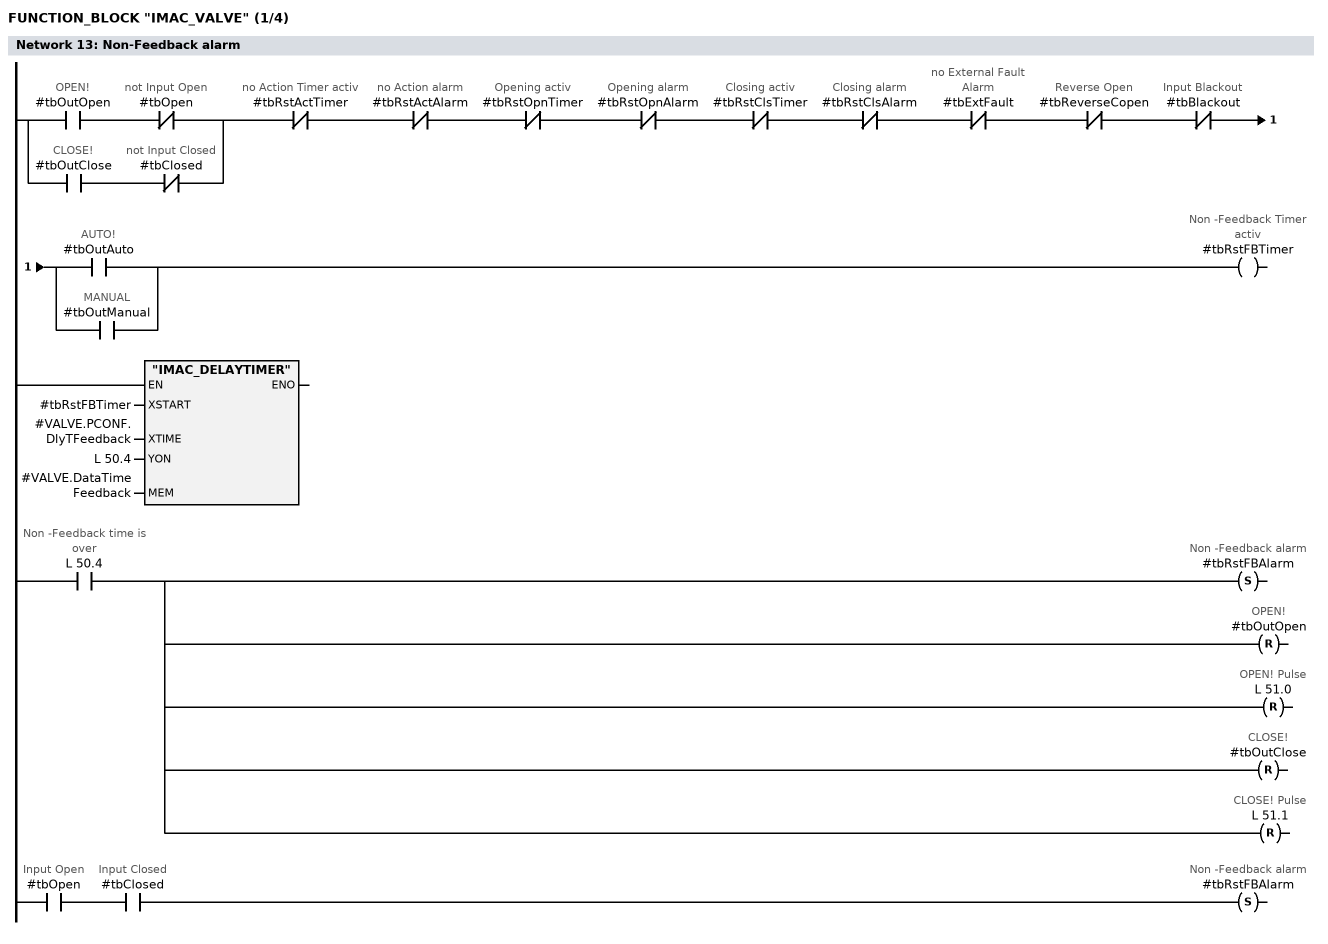
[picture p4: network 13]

      O(    ;
      U     #tbOutOpen; // OPEN!
      UN    #tbOpen; // not Input Open
      )     ;
      O(    ;
      U     #tbOutClose; // CLOSE!
      UN    #tbClosed; // not Input Closed
      )     ;
      UN    #tbRstActTimer; // no Action Timer activ
      UN    #tbRstActAlarm; // no Action alarm
      UN    #tbRstOpnTimer; // Opening activ
      UN    #tbRstOpnAlarm; // Opening alarm
      UN    #tbRstClsTimer; // Closing activ
      UN    #tbRstClsAlarm; // Closing alarm
      UN    #tbExtFault; // no External Fault Alarm
      UN    #tbReverseCopen; // Reverse Open
      UN    #tbBlackout; // Input Blackout
      U(    ;
      O     #tbOutAuto; // AUTO!
      O     #tbOutManual; // MANUAL
      )     ;
      =     #tbRstFBTimer; // Non -Feedback Timer activ

//Non -Feedbackn timer
      CALL "IMAC_DELAYTIMER" (
           XSTART                   := #tbRstFBTimer,// Non -Feedback Timer activ
           XTIME                    := #VALVE.PCONF.DlyTFeedback,
           YON                      := L     50.4,
           MEM                      := #VALVE.DataTimeFeedback);

      U     L     50.4; // Non -Feedback time is over
      S     #tbRstFBAlarm; // Non -Feedback alarm
      R     #tbOutOpen; // OPEN!
      R     L     51.0; // OPEN! Pulse
      R     #tbOutClose; // CLOSE!
      R     L     51.1; // CLOSE! Pulse
      U     #tbOpen; // Input Open
      U     #tbClosed; // Input Closed
      S     #tbRstFBAlarm; // Non -Feedback alarm
NETWORK
TITLE =Automatic States
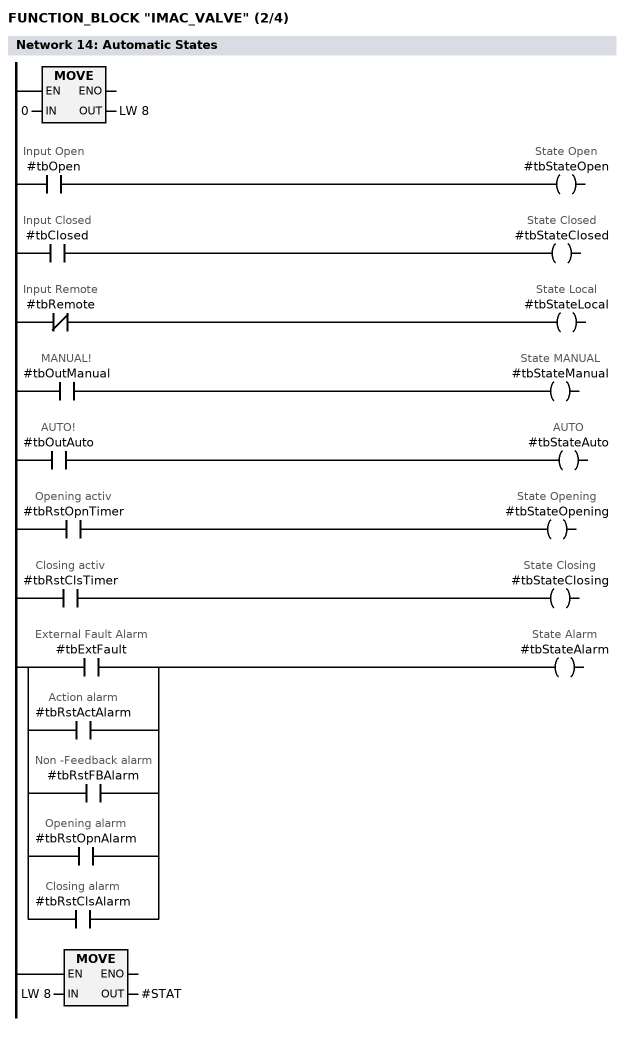
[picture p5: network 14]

      L     0;
      T     LW     8;

      U     #tbOpen; // Input Open
      =     #tbStateOpen; // State Open
      U     #tbClosed; // Input Closed
      =     #tbStateClosed; // State Closed
      UN    #tbRemote; // Input Remote
      =     #tbStateLocal; // State Local
      U     #tbOutManual; // MANUAL!
      =     #tbStateManual; // State MANUAL
      U     #tbOutAuto; // AUTO!
      =     #tbStateAuto; // AUTO
      U     #tbRstOpnTimer; // Opening activ
      =     #tbStateOpening; // State Opening
      U     #tbRstClsTimer; // Closing activ
      =     #tbStateClosing; // State Closing
      O     #tbExtFault; // External Fault Alarm
      O     #tbRstActAlarm; // Action alarm
      O     #tbRstFBAlarm; // Non -Feedback alarm
      O     #tbRstOpnAlarm; // Opening alarm
      O     #tbRstClsAlarm; // Closing alarm
      =     #tbStateAlarm; // State Alarm

      L     LW     8; // State To Automatic
      T     #STAT;
NETWORK
TITLE =Lock/ Emergency Off
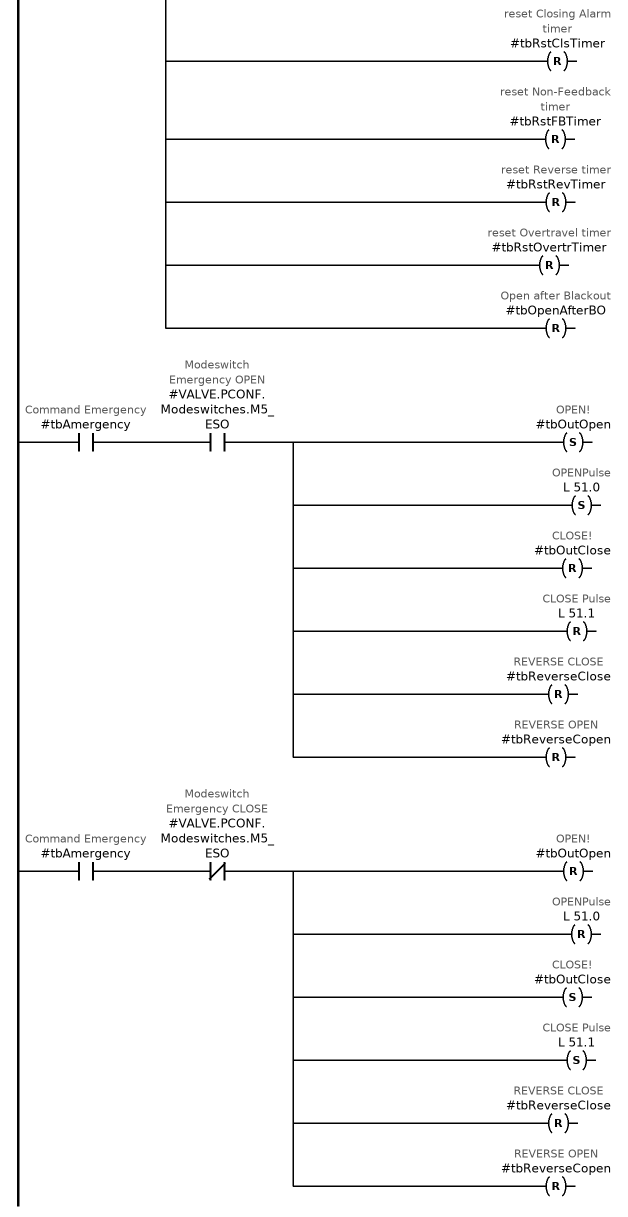
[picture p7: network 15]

      U     #tbLock; //Command LOCK
      U(    ;
      O     #tbOutAuto; // AUTO!
      O     #tbOutManual; // MANUAL
      )     ;
      R     #tbRstActAlarm; // reset Action Alarm
      R     #tbRstOpnAlarm; // reset Opening Alarm
      R     #tbRstClsAlarm; // reset Closing Alarm
      R     #tbRstFBAlarm; // reset Non-Feedback Alarm
      R     #tbRstActTimer; // reset Action Timer
      R     #tbRstOpnTimer; // reset Opening Alarm timer
      R     #tbRstClsTimer; // reset Closing Alarm timer
      R     #tbRstFBTimer; // reset Non-Feedback timer
      R     #tbRstRevTimer; // reset Reverse timer
      R     #tbRstOvertrTimer; // reset Overtravel timer
      R     #tbOpenAfterBO; // Open after Blackout

      U     #tbLock; //Command LOCK
      U     #VALVE.PCONF.Modeswitches.M4_LockInput; //Modeswitch Lock blocks Commands
      U(    ;
      O     #tbOutAuto; // AUTO!
      O     #tbOutManual; // MANUAL
      )     ;
      R     #tbOutOpen; // OPEN!
      R     L     51.0; // OPENPulse
      R     #tbOutClose; // CLOSE!
      R     L     51.1; // CLOSE Pulse
      R     #tbReverseClose; // REVERSE CLOSE
      R     #tbReverseCopen; // REVERSE OPEN

//---- Emergency OPEN / CLOSE
      U     #tbAmergency; //Command Emergency
      R     #tbRstActTimer; // reset Action Timer
      R     #tbRstOpnTimer; // reset Opening Alarm timer
      R     #tbRstClsTimer; // reset Closing Alarm timer
      R     #tbRstFBTimer; // reset Non-Feedback timer
      R     #tbRstRevTimer; // reset Reverse timer
      R     #tbRstOvertrTimer; // reset Overtravel timer
      R     #tbOpenAfterBO; // Open after Blackout

      U     #tbAmergency; //Command Emergency
      U     #VALVE.PCONF.Modeswitches.M5_ESO; //Modeswitch Emergency OPEN
      S     #tbOutOpen; // OPEN!
      S     L     51.0; // OPENPulse
      R     #tbOutClose; // CLOSE!
      R     L     51.1; // CLOSE Pulse
      R     #tbReverseClose; // REVERSE CLOSE
      R     #tbReverseCopen; // REVERSE OPEN

      U     #tbAmergency; // Command Emergency
      UN    #VALVE.PCONF.Modeswitches.M5_ESO; // Modeswitch Emergency CLOSE
      R     #tbOutOpen; // OPEN!
      R     L     51.0; // OPENPulse
      S     #tbOutClose; // CLOSE!
      S     L     51.1; // CLOSE Pulse
      R     #tbReverseClose; // REVERSE CLOSE
      R     #tbReverseCopen; // REVERSE OPEN
NETWORK
TITLE =Output
//OUTPUT VOPN
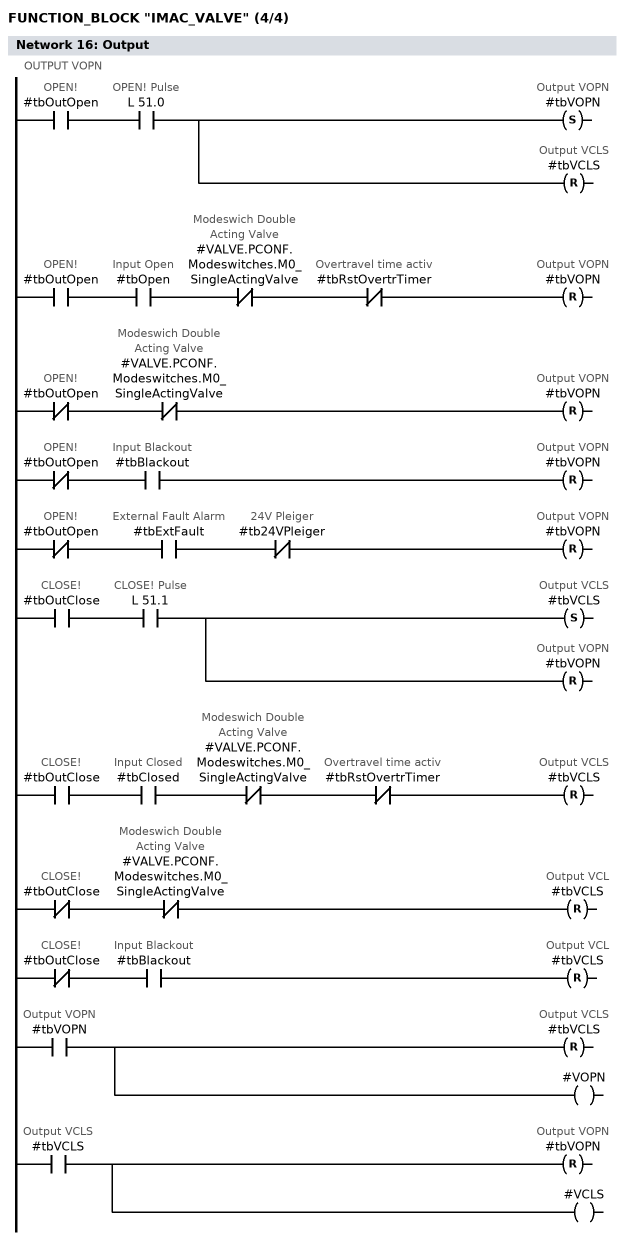
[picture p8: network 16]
      U     #tbOutOpen; // OPEN!
      U     L     51.0; // OPEN! Pulse
      S     #tbVOPN; // Output VOPN
      R     #tbVCLS; // Output VCLS

// -------Reseting Output VOPN by  Double Acting Valve-----
      U     #tbOutOpen; // OPEN!
      U     #tbOpen; // Input Open
      UN    #VALVE.PCONF.Modeswitches.M0_SingleActingValve; // Modeswich Double Acting Valve
      UN    #tbRstOvertrTimer; // Overtravel time activ
      R     #tbVOPN; // Output VOPN

      UN    #tbOutOpen; // OPEN!
      UN    #VALVE.PCONF.Modeswitches.M0_SingleActingValve; // Modeswich Double Acting Valve
      R     #tbVOPN; // Output VOPN

// -------Reseting Output VOPN by  Blackout -----
      UN    #tbOutOpen; // OPEN!
      U     #tbBlackout; // Input Blackout
      R     #tbVOPN; // Output VOPN

// -------Reseting Output VOPN Double Acting Valve  Pleiger-----
// Rücksetzen des VOPN Ausgangs nur wenn
// Externer Fehler ansteht und 24 Volt ausgefallen sind

      UN    #tbOutOpen; // OPEN!
      U     #tbExtFault; // External Fault Alarm
      UN    #tb24VPleiger; // 24V Pleiger
      R     #tbVOPN; // Output VOPN

//OUTPUT VCLS
      U     #tbOutClose; // CLOSE!
      U     L     51.1; // CLOSE! Pulse
      S     #tbVCLS; // Output VCLS
      R     #tbVOPN; // Output VOPN

// -------Reseting Output VCLS Double Acting Valve-----
      U     #tbOutClose; // CLOSE!
      U     #tbClosed; // Input Closed
      UN    #VALVE.PCONF.Modeswitches.M0_SingleActingValve; // Modeswich Double Acting Valve
      UN    #tbRstOvertrTimer; // Overtravel time activ
      R     #tbVCLS; // Output VCLS

      UN    #tbOutClose; // CLOSE!
      UN    #VALVE.PCONF.Modeswitches.M0_SingleActingValve; // Modeswich Double Acting Valve
      R     #tbVCLS; // Output VCL

// -------Reseting Output VCLS by  Blackout -----
      UN    #tbOutClose; // CLOSE!
      U     #tbBlackout; // Input Blackout
      R     #tbVCLS; // Output VCL

//SET OUTPUTS
      U     #tbVOPN; // Output VOPN
      R     #tbVCLS; // Output VCLS
      =     #VOPN;
      U     #tbVCLS; // Output VCLS
      R     #tbVOPN; // Output VOPN
      =     #VCLS;
NETWORK
TITLE =Combinate States
//----Alarms----
      U     #tbLock; //Command LOCK
      U(    ;
      O     #tbOutAuto; // AUTO!
      O     #tbOutManual; // MANUAL
      )     ;
      L     7;
      SPB   COD1;
      U     #tbAmergency; //Command Emergency
      L     8;
      SPB   COD1;

      UN    #tbRstActAlarm; // Action Alarm
      UN    #tbRstOpnAlarm; // Opening Alarm
      UN    #tbRstClsAlarm; // Closing Alarm
      UN    #tbRstFBAlarm; // Non-Feedback Alarm
      UN    #tbExtFault; // External Fault Alarm
      L     1; // Normal
      SPB   COD1;
      U     #tbExtFault; // External Fault Alarm
      L     2;
      SPB   COD1;
      U     #tbRstActAlarm; // Action Alarm
      L     3;
      SPB   COD1;
      U     #tbRstOpnAlarm; // Opening Alarm
      L     4;
      SPB   COD1;
      U     #tbRstClsAlarm; // Closing Alarm
      L     5;
      SPB   COD1;
      U     #tbRstFBAlarm; // Non-Feedback Alarm
      L     6; //
      SPB   COD1;
      L     0; //Undefined
COD1: T     LW    10; //States to OS

//----Status----
      UN    #tbOpen; //Input Open
      UN    #tbClosed; //Input Close
      UN    #tbStateOpening; //Opening
      UN    #tbStateClosing; //Closing
      L     5; // UNDEFINED POSITION
      SPB   COD2;
      U     #tbOpen; //Input Open
      L     1; //OPENED
      SPB   COD2;
      U     #tbClosed; //Input Close
      L     2; //CLOSED
      SPB   COD2;
      U     #tbStateOpening; // State opening
      L     3; // OPENING
      SPB   COD2;
      U     #tbStateClosing; // State closing
      L     4; // CLOSING
      SPB   COD2;
      L     0; //Undefined
COD2: T     LW    12; //States to OS

      U     #tbLocal; //Local?
      L     256;
      SPB   COD3;
      U     #tbStateManual; //Manual?
      L     512;
      SPB   COD3;
      U     #tbOutAuto; // AUTO?
      L     1024;
      SPB   COD3;
      L     0;
COD3: L     LW    12; //Basic states
      +I    ;
      T     LW    12; //Combinate states to OS


NETWORK
TITLE = Store States in Record

      L     0; // Reset Commands OS
      T     #VALVE.CmdOS;
      T     #OSCOM; // Write Reset Back to I/O interface  added: 20060619 /Ho
      L     LW    10;
      T     #VALVE.AlarmOS; // Alarms to OS
      T     #OSALARM;
      L     LW    12;
      T     #VALVE.StatusOS; // States to OS
      T     #OSSTAT;
      L     LW    14;
      T     #VALVE.Status1; // Status stored
      L     LW    16;
      T     #VALVE.Status2; // Status stored
NETWORK
TITLE =Write record

      CALL "BLKMOV" (
           SRCBLK                   := #VALVE,
           RET_VAL                  := #siFailWR,
           DSTBLK                   := #P_currentRecord);

END_FUNCTION_BLOCK

